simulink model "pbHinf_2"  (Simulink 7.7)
settings: Solver=ode45  StartTime=0.0  StopTime=10.0  RelTol=1e-3
libraries: cstblocks x2

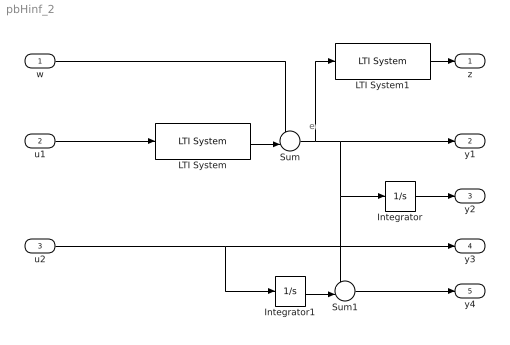
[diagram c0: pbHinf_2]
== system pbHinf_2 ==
  note: e
  w : Inport
  u1 : Inport  Port=2
  u2 : Inport  Port=3
  Integrator : Integrator
  Integrator1 : Integrator
  LTI System : cstblocks/LTI System  SystemSampleTime=-1  sys=G  IC=[]
  LTI System1 : cstblocks/LTI System  SystemSampleTime=-1  sys=W1  IC=[]
  Sum : Sum  Inputs=+-|
  Sum1 : Sum  Inputs=+-|
  z : Outport
  y1 : Outport  Port=2
  y2 : Outport  Port=3
  y3 : Outport  Port=4
  y4 : Outport  Port=5
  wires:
  LTI System/1 -> Sum/2
  w/1 -> Sum/1
  u1/1 -> LTI System/1
  LTI System1/1 -> z/1
  Sum/1 -> LTI System1/1, y1/1, Integrator/1, Sum1/1
  Integrator/1 -> y2/1
  u2/1 -> y3/1, Integrator1/1
  Integrator1/1 -> Sum1/2
  Sum1/1 -> y4/1
